PROGRAM MAIN
VAR
	Ramp: LREAL;	
	Sinus: LREAL;
	
	t: UINT;
	Ts: UINT;	
	phi: LREAL;
END_VAR

// ramp
Ramp:=Ramp+0.002;

IF (Ramp > 1.0) THEN
	Ramp:=-1.0;
END_IF

// sinus
t := t + 1;
Ts:=128*10;

IF (t>=2*Ts) THEN
	t:=t-2*Ts;
END_IF

Sinus:=COS(PI*t/Ts);

END_PROGRAM
